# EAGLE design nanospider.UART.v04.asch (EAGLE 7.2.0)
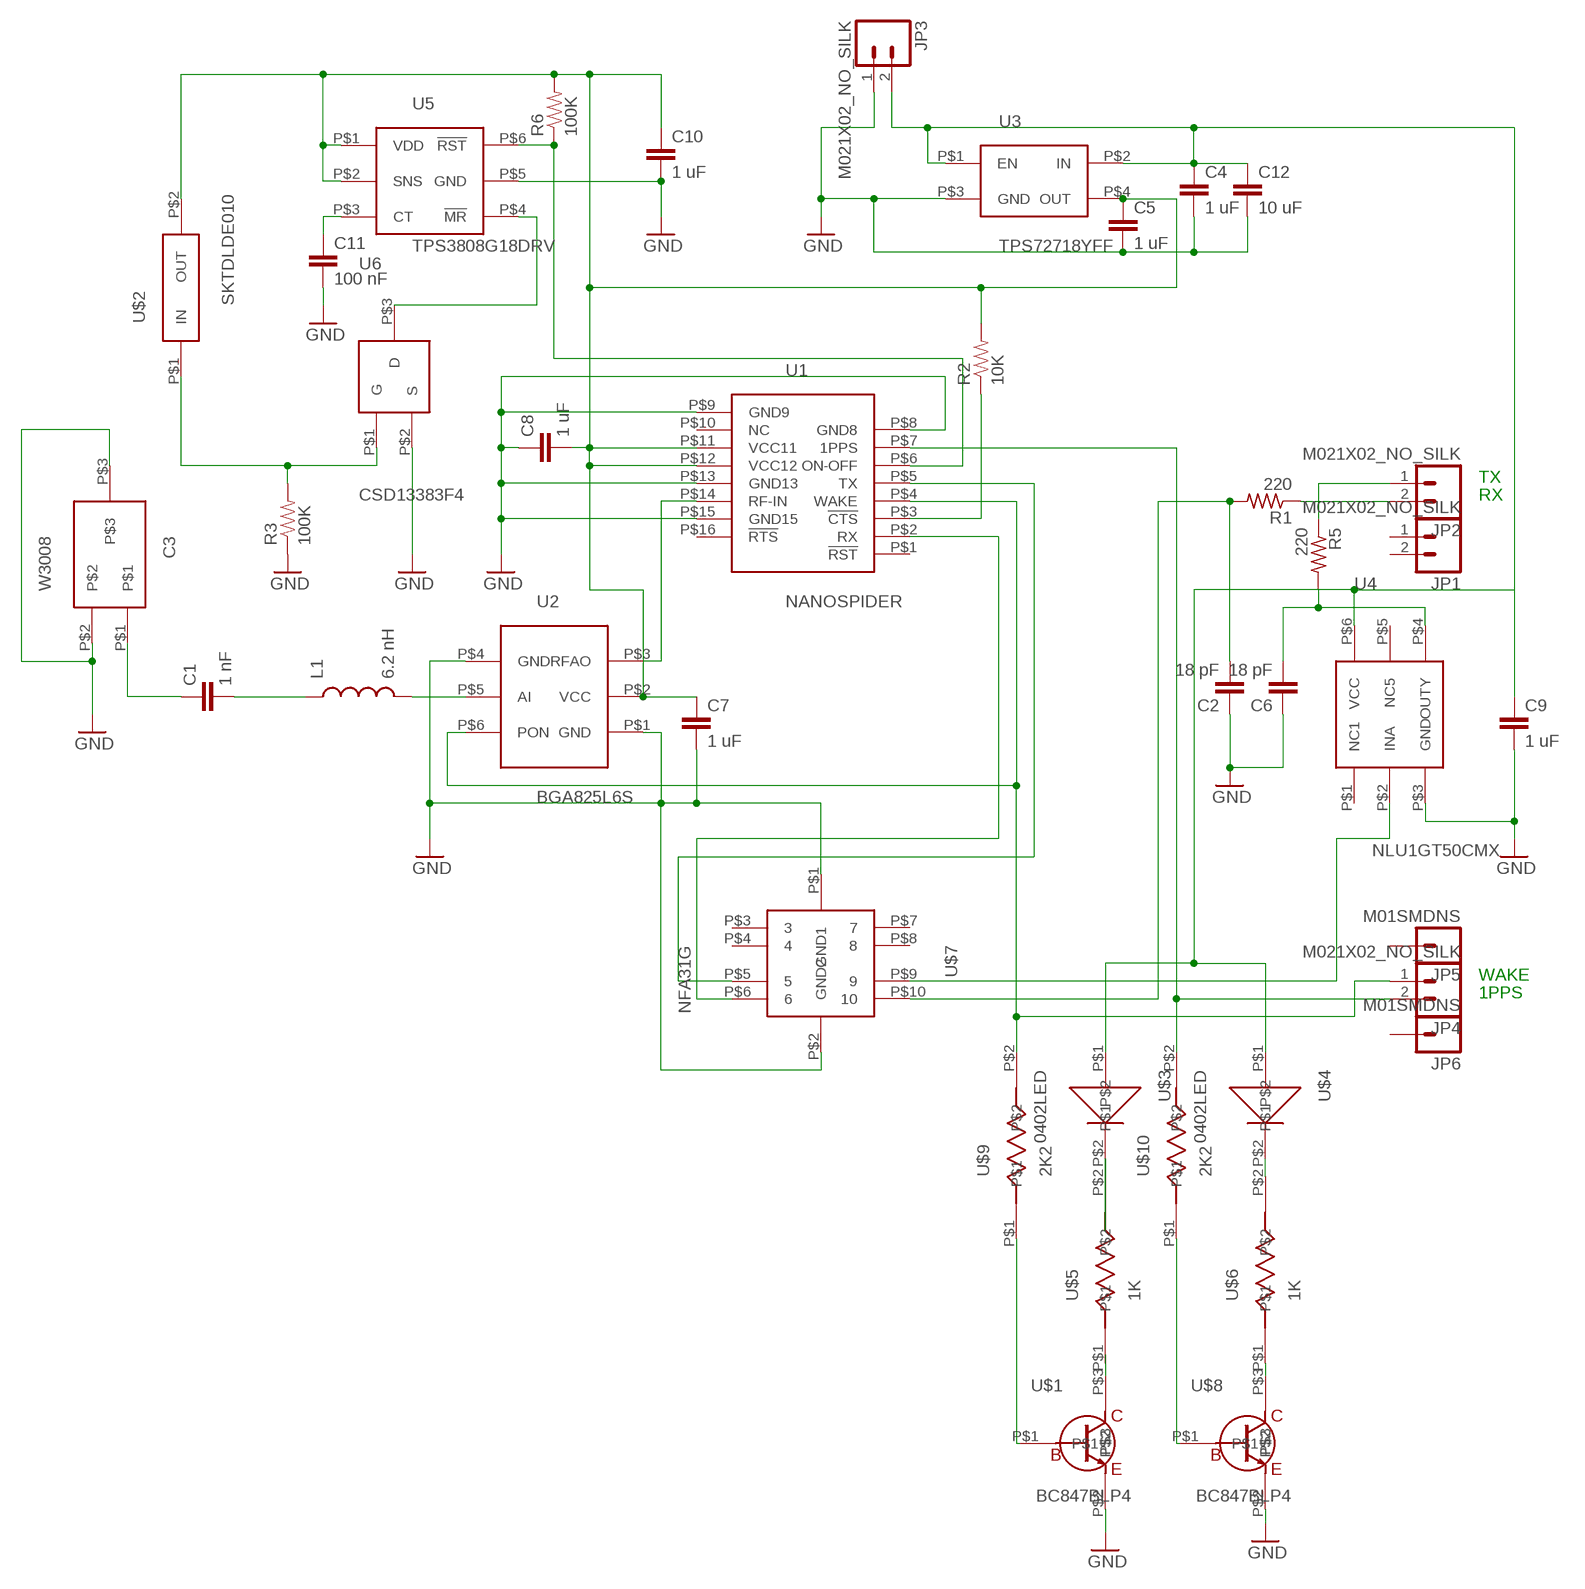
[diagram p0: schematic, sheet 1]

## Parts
C1  1 nF  0402CAP.KW  [0402-CAP]
C2  18 pF  C-EUC0402  [C0402]
C3  W3008  [W008]
C4  1 uF  0402CAP.KW  [0402-CAP]
C5  1 uF  0402CAP.KW  [0402-CAP]
C6  18 pF  C-EUC0402  [C0402]
C7  1 uF  0402CAP.KW  [0402-CAP]
C8  1 uF  0402CAP.KW  [0402-CAP]
C9  1 uF  0402CAP.KW  [0402-CAP]
C10  1 uF  0402CAP.KW  [0402-CAP]
C11  100 nF  0402CAP.KW  [0402-CAP]
C12  10 uF  0402CAP.KW  [0402-CAP]
JP1  M021X02_NO_SILK  [1X02_NO_SILK]
JP2  M021X02_NO_SILK  [1X02_NO_SILK]
JP3  M021X02_NO_SILK  [1X02_NO_SILK]
JP4  M021X02_NO_SILK  [1X02_NO_SILK]
JP5  M01SMDNS  [1X01NS]
JP6  M01SMDNS  [1X01NS]
L1  6.2 nH  INDUCTOR0402  [C0402]
R1  220  R-US_R0402  [R0402]
R2  10K  0402RES.KW  [0402-RES]
R3  100K  0402RES.KW  [0402-RES]
R5  220  R-US_R0402  [R0402]
R6  100K  0402RES.KW  [0402-RES]
U1  NANOSPIDER  [NANOSPIDER]
U2  BGA825L6S  [BGA825L6S]
U3  TPS72718YFF  [YFF0004]
U4  NLU1GT50CMX  [ULLGA6]
U5  TPS3808G18DRV  [PWSON-N6]
U6  CSD13383F4  [CSD13383F4]
U$1  BC847BLP4  [DFN1006]
U$2  SKTDLDE010  [SKTDLDE010]
U$3  0402LED  [0402LED]
U$4  0402LED  [0402LED]
U$5  1K  0402RESISTOR  [0402RESISTOR]
U$6  1K  0402RESISTOR  [0402RESISTOR]
U$7  NFA31G  [NFA31G]
U$8  BC847BLP4  [DFN1006]
U$9  2K2  0402RESISTOR  [0402RESISTOR]
U$10  2K2  0402RESISTOR  [0402RESISTOR]

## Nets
GND: C2.1 C3.P$2 C3.P$3 C4.2 C5.2 C6.1 C7.2 C8.1 C9.2 C10.2 C11.2 C12.2 JP3.1 R3.1 U1.P$8(GND8) U1.P$9(GND9) U1.P$13(GND13) U1.P$15(GND15) U2.P$1(GND) U2.P$4(GNDRF) U3.P$3(GND) U4.P$3(GND) U5.P$5(GND) U6.P$2(S) U$1.P$2 U$7.P$1(GND1) U$7.P$2(GND2) U$8.P$2
N$1: C1.1 C3.P$1
N$2: C1.2 L1.1
N$3: L1.2 U2.P$5(AI)
N$4: U1.P$14(RF-IN) U2.P$3(AO)
N$6: JP2.2 R1.1
N$7: U1.P$2(RX) U$7.P$6
N$8: U4.P$2(INA) U$7.P$9
N$9: C2.2 R1.2 U$7.P$10
N$10: C4.1 C9.1 C12.1 JP3.2 U3.P$1(EN) U3.P$2(IN) U4.P$6(VCC) U$3.P$1 U$4.P$1
N$11: C5.1 C7.1 C8.2 C10.1 R2.2 R6.2 U1.P$11(VCC11) U1.P$12(VCC12) U2.P$2(VCC) U3.P$4(OUT) U5.P$1(VDD) U5.P$2(SNS) U$2.P$2(OUT)
N$12: R3.2 U6.P$1(G) U$2.P$1(IN)
N$13: C11.1 U5.P$3(CT)
N$14: JP2.1 R5.1
N$15: U1.P$5(TX) U$7.P$5
N$16: U$1.P$1 U$9.P$1
N$17: R6.1 U1.P$6(ON-OFF) U5.P$6(!RST)
N$18: U5.P$4(!MR) U6.P$3(D)
N$19: U$1.P$3 U$5.P$1
N$20: U$3.P$2 U$5.P$2
N$21: U$8.P$1 U$10.P$1
N$22: JP4.1 U1.P$4(WAKE) U2.P$6(PON) U$9.P$2
N$23: U$6.P$1 U$8.P$3
N$27: C6.2 R5.2 U4.P$4(OUTY)
N$29: JP4.2 U1.P$7(1PPS) U$10.P$2
N$32: U$4.P$2 U$6.P$2
N$33: R2.1 U1.P$3(!CTS)
Unconnected: JP1.1 JP1.2 JP5.1 JP6.1 U1.P$1(!RST) U1.P$10(NC) U1.P$16(!RTS) U4.P$1(NC1) U4.P$5(NC5) U$7.P$3 U$7.P$4 U$7.P$7 U$7.P$8

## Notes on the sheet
- TX
- RX
- WAKE
- 1PPS

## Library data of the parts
C1 C4 C5 C7-C12 = SparkFun-Capacitors:0402CAP.KW
C2 C6 = rcl:C-EU: CAPACITOR, European symbol
C3 = Kris:W3008: W3008 2.4 GHz ceramic antenna
JP1-JP4 = SparkFun-Connectors:M02: Standard 2-pin 0.1" header. Use with
JP5 JP6 = SparkFun-Connectors:M01: Header 1
L1 = SparkFun-Passives:INDUCTOR: Inductors
R1 R5 = rcl:R-US_: RESISTOR, American symbol
R2 R3 R6 = SparkFun-Resistors:0402RES.KW
U1 = Kris:NANOSPIDER: Origin Nano Spider 4 mm x 4 mm GPS module
U2 = Kris:BGA825L6S: Infineon BGA 825L6S 1.8 V BGA amplifier for GNSS
U3 = Kris:TPS72718YFF: TI's TPS72718YFF 1.8 V RF voltage regulator
U4 = Kris:NLU1GT50CMX: NLU1GT50CMX non-inverting buffer
U5 = Kris:TPS3808G18DRV: PWSON-N6 package for TI's TPS3808G18DRV Supervisory Circuit
U6 = Kris:CSD13383F4: TI's CSD13383F4 12V N-Channel FemtoFet MOSFET
U$1 U$8 = Kris:BC847BLP4: DFN1006 package for BC847BLP4 45 V small signal NPN transistor
U$2 = Kris:SKTDLDE010: ALPS SKTDLDE010 side-mount tac switch
U$3 U$4 = Kris:0402LED: 0402led
U$5 U$6 U$9 U$10 = Kris:0402RESISTOR: 0402 resistor
U$7 = Kris:NFA31G

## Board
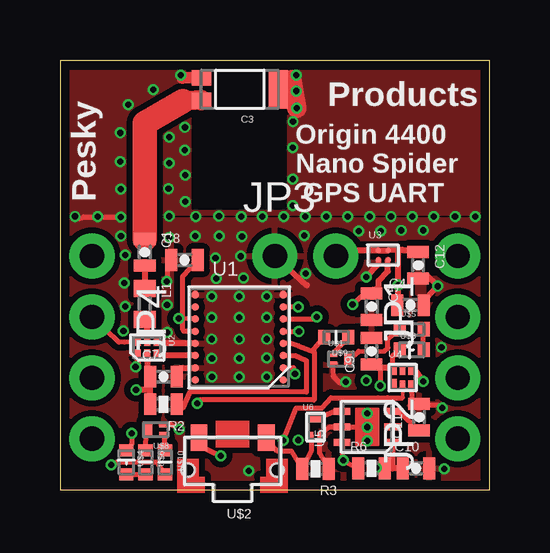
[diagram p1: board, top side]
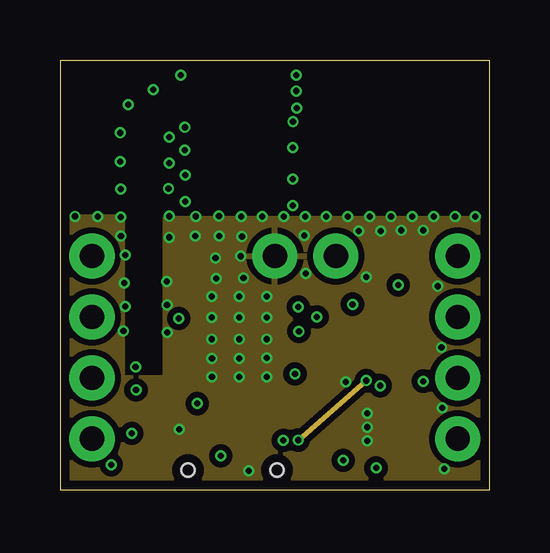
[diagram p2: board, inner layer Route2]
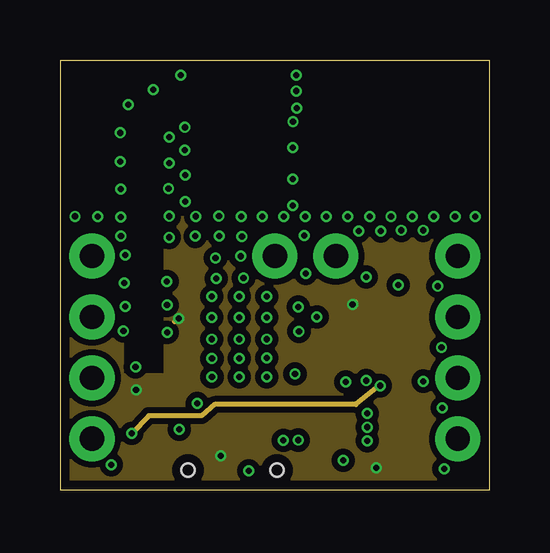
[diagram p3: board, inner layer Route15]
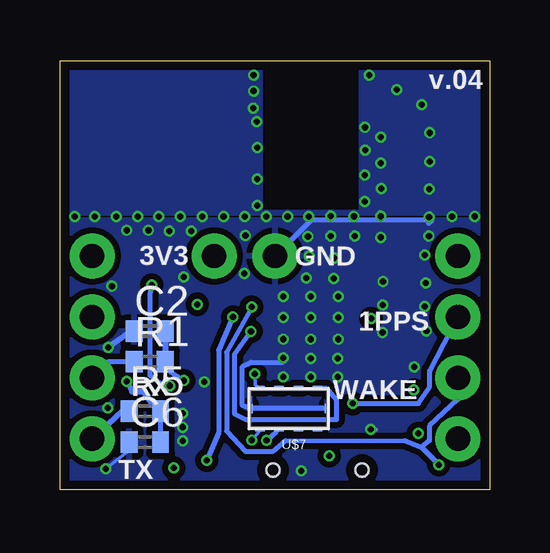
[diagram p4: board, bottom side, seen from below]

Size 17.91 x 17.9 mm. Coordinates in mm from the lower left corner, seen from the top.
Outline: 0,0 17.91,0 17.91,17.9 0,17.9 0,0
Copper layers (1*2*15*16): Top 0.035559375mm / dielectric 0.17018125mm / Route2 0.01778125mm / dielectric 47mil / Route15 0.01778125mm / dielectric 0.17018125mm / Bottom 0.035559375mm
Design rules "OSHPark-4layer *": minimum track width 5mil, minimum drill 10mil, track to track 5mil, track to pad 5mil, pad to pad 5mil, via to via 5mil, smd to smd 5mil, copper to edge 15mil, drill to drill 6mil, minimum pad ring 4mil, minimum via ring 4mil, stop-mask expansion 4mil, vias tented up to drill 20mil, thermal gap 10mil

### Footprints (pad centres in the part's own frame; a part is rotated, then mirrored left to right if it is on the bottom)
0402-CAP = smd 0.5 x 0.9: 1 -0.55,0; 2 0.55,0
C0402 = smd 0.7 x 0.9: 1 -0.65,0; 2 0.65,0
W008 = smd 0.8 x 0.65: P$1 1.6,0.475; P$2 1.6,-0.475 | smd 0.8 x 1.6: P$3 -1.6,0
1X02_NO_SILK = drill 1.016 pad 1.88: 1 0,0; 2 2.54,0
1X01NS = drill 1.016 pad 1.88: 1 0,0
R0402 = smd 0.7 x 0.9: 1 -0.65,0; 2 0.65,0
0402-RES = smd 0.5 x 0.9: 1 -0.55,0; 2 0.55,0
NANOSPIDER = smd 0.305 x 0.305: P$1 1.829,-1.778; P$2 1.829,-1.27; P$3 1.829,-0.762; P$4 1.829,-0.254; P$5 1.829,0.254; P$6 1.829,0.762; P$7 1.829,1.27; P$8 1.829,1.778; P$9 -1.829,1.778; P$10 -1.829,1.27; P$11 -1.829,0.762; P$12 -1.829,0.254; P$13 -1.829,-0.254; P$14 -1.829,-0.762; P$15 -1.829,-1.27; P$16 -1.829,-1.778
BGA825L6S = smd 0.3 x 0.25: P$1 0.225,-0.4; P$2 0.225,0; P$3 0.225,0.4; P$4 -0.225,0.4; P$5 -0.225,0; P$6 -0.225,-0.4
YFF0004 = smd 0.23 x 0.23: P$1 -0.2,0.2; P$2 0.2,0.2; P$3 -0.2,-0.2; P$4 0.2,-0.2
ULLGA6 = smd 0.22 x 0.53: P$1 -0.35,-0.325 | smd 0.22 x 0.48: P$2 0,-0.35; P$3 0.35,-0.35; P$4 0.35,0.35; P$5 0,0.35; P$6 -0.35,0.35
PWSON-N6 = smd 0.3 x 0.7: P$1 -0.65,-1.05; P$2 0,-1.05; P$3 0.65,-1.05; P$4 0.65,1.05; P$5 0,1.05; P$6 -0.65,1.05
CSD13383F4 = smd 0.15 x 0.25: P$1 -0.175,-0.325; P$2 0.175,-0.325 | smd 0.5 x 0.25: P$3 0.005,0.315
DFN1006 = smd 0.4 x 0.25: P$1 -0.35,0.225; P$2 -0.35,-0.225 | smd 0.4 x 0.7: P$3 0.35,0
SKTDLDE010 = smd 0.7 x 1.1: P$1 -1.4,-0.975; P$2 1.4,-0.975 | hole 0.55: -1.85,0.375; 1.85,0.375
0402LED = smd 0.5 x 0.6: P$1 -0.5,0; P$2 0.5,0
0402RESISTOR = smd 0.5 x 0.6: P$1 -0.5,0; P$2 0.5,0
NFA31G = smd 0.2 x 0.4: P$1 -1.6,0; P$2 1.6,0 | smd 0.4 x 0.2: P$3 -0.4,-0.85; P$4 0.4,-0.85; P$5 -1.2,-0.85; P$6 1.2,-0.85; P$7 -1.2,0.85; P$8 -0.4,0.85; P$9 0.4,0.85; P$10 1.2,0.85

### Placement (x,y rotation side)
C1  3.53,9.91 270 top
C2  14.17,6.6 0 bottom
C3  7.49,16.7 180 top
C4  14.6,7.7 0 top
C5  12.98,7.64 270 top
C6  14.38,1.98 0 bottom
C7  4.31,4.71 0 top
C8  5.19,9.58 0 top
C9  12.98,5.77 90 top
C10  14.83,0.89 0 top
C11  14.96,3.02 90 top
C12  14.92,9.35 270 top
JP1  16.57,7.2 90 top
JP2  16.57,2.12 90 top
JP3  8.95,9.74 0 top
JP4  1.33,7.2 270 top
JP5  1.33,2.12 0 top
JP6  1.33,9.74 0 top
L1  3.53,7.74 270 top
R1  14.17,5.33 0 bottom
R2  4.31,3.56 180 top
R3  10.65,0.87 180 top
R5  14.38,3.28 0 bottom
R6  12.98,0.89 0 top
U1  7.47,6.35 0 top
U2  3.63,5.92 270 top
U3  13.47,9.78 0 top
U4  14.27,4.67 0 top
U5  12.8,2.62 90 top
U6  10.64,2.62 0 top
U$1  11.7,5.44 0 top
U$2  7.19,1.19 180 top
U$3  14.65,5.83 0 top
U$4  2.76,1.14 270 top
U$5  14.65,6.68 0 top
U$6  3.57,1.14 270 top
U$7  8.38,3.38 180 bottom
U$8  3.99,2.5 180 top
U$9  11.5,6.36 180 top
U$10  4.38,1.14 270 top

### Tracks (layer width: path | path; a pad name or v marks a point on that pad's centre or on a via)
GND  (via drill 0.25)
  Top 0.152: U4.P$3 14.65,4.04 | v16,0.86 16.18,0.86
  Top 0.203: 4.07,6.16 U2.P$4 | 0.79,11.3 0.98,11.37 v2.54,11.37 | C8.1 4.48,9.37 4.47,9.07 4.48,8.7 v4.46,8.68 | C4.2 15.13,7.73 15.01,7.75 | R3.1 10.82,1.52 U6.P$2 10.82,2.31 11.25,2.62 U5.P$5 | 11.5,2.59 U5.P$5 | 14.65,4.04 14.65,3.53 | 14.65,3.53 C11.2 | 14.65,3.53 15.93,3.53 v15.93,3.4 | U5.P$5 12.79,2.62 v12.8,2.61 | U$1.P$2 11.38,4.72 11.65,4.46 11.87,4.46 v11.91,4.5 | 3.24,5.16 v3.15,5.11 | U$8.P$2 4.61,2.72 v4.97,2.51
  Top 0.254: U1.P$13 4.32,6.1 4.07,6.16 | 10.29,8.52 JP3.1 | U1.P$15 5.59,5.05 4.97,5.05 4.95,4.83 C7.2 | 15.01,7.75 v15.75,8.48 15.29,8.94 | U2.P$1 3.24,5.67 3.24,5.16 | U3.P$3 13.27,9.4 v12.76,8.86
  Top 0.406: 5.11,17.16 v5.02,17.28
  Top 0.508: C3.P$2 5.11,17.16
  Top 0.813: C3.P$3 9.66,17.11 v9.87,15.9
  Bottom 0.152: C6.1 15,1.66 v16,0.86
  Bottom 0.203: 9.12,9.63 JP3.1 7.44,11.25 2.41,11.25 2.56,11.1 v2.54,11.37 | U$7.P$1 U$7.P$2 10.31,3.51 10.31,5.13 9.96,5.31 8.64,5.31 v8.61,5.49 | v15.93,3.4 15.95,3.38 | v11.91,4.5 11.92,4.51 v11.92,4.5 | v4.97,2.51 4.94,2.49 4.78,2.5
  Bottom 0.254: C2.1 15.14,6.48 v15.89,5.93 | v12.76,8.86 12.69,8.86
  other vias: 0.62,11.4 4.55,11.4 6.62,11.4 7.54,11.39 9.32,11.39 11.1,11.39 11.99,11.39 15.57,11.39 17.3,11.39 4.46,7.69 4.48,6.55 2.68,8.63 2.64,6.61 10.19,10.59 10.24,9.02 6.32,8.05 7.47,8.05 8.61,8.05 6.32,7.19 6.32,6.27 6.33,5.46 7.47,7.19 8.61,7.19 7.47,6.27 8.61,6.27 7.47,5.47 2.72,9.78 2.72,7.65 10.21,11.39 3.89,16.69 2.84,16.05 2.51,14.88 2.51,13.67 2.52,12.53 4.52,12.55 4.55,13.61 4.55,14.71 5.21,15.11 5.2,14.15 5.22,13.11 5.22,12.01 8.43,11.39 9.7,11.84 9.7,12.96 9.69,14.27 9.71,15.35 9.85,17.28 9.85,16.63 5.66,11.4 7.87,0.78 12.8,3.17 12.8,2.04 6.33,4.71 7.47,4.71 8.61,4.71 4.55,10.52 2.54,10.58 1.58,11.38 12.9,11.39 13.79,11.39 14.68,11.38 16.46,11.39 5.64,10.57 6.63,10.57 7.58,10.55 6.48,9.66 6.5,8.81 7.52,9.73 7.65,8.83 12.45,10.79 13.36,10.79 14.23,10.82 15.13,10.82
  pour Top (isolate 0.254): 17.91,11.28 17.97,-0.02 0.04,-0.02 -0.03,11.3
  pour Bottom (isolate 0.254): -0.03,11.28 17.83,11.28 17.95,-0.02 0.01,-0.02
  pour Route2 (isolate 0.254): 0,11.38 2.59,11.4 2.59,4.67 4.39,4.7 4.39,11.33 17.91,11.33 17.87,-0.02 -0.06,-0.02 -0.03,11.38
  pour Top (isolate 0.254): 0,17.93 5.46,17.93 5.46,11.66 9.46,11.66 9.46,17.93 17.91,17.93 17.91,11.43 0,11.43
  pour Bottom (isolate 0.254): 0,17.93 5.46,17.93 5.46,11.66 9.46,11.66 9.46,17.93 17.91,17.93 17.91,11.43 0,11.43
N$1
  Top 0.813: 5.11,16.21 5.88,16.26 C3.P$1
  Top 1.016: C1.1 3.53,15.29 5.11,16.21
N$2
  Top 0.254: C1.2 L1.1
N$3
  Top 0.203: 3.63,6.88 L1.2
  Top 0.254: U2.P$5 3.63,6.88
N$4
  Top 0.254: U2.P$3 4.19,5.59 4.37,5.59 U1.P$14
N$6
  Bottom 0.203: 15.11,5.33 15.9,5.33 JP2.2
  Bottom 0.254: R1.1 15.11,5.33
N$7  (via drill 0.25)
  Top 0.203: v9.79,4.83 9.78,4.98 9.73,5.08 U1.P$2
  Bottom 0.152: U$7.P$6 9.79,4.38 v9.79,4.83
N$8  (via drill 0.25)
  Top 0.152: U4.P$2 14.28,3.84
  Top 0.203: v9.31,2.06 9.84,3.4 10.92,3.4 11.3,3.83 13.25,3.83 13.64,3.84 14.28,3.84
  Bottom 0.152: U$7.P$9 8.85,2.43 v9.31,2.06
  Bottom 0.203: v9.31,2.06 8.89,2.43
N$9  (via drill 0.25)
  Route2 0.203: v9.93,2.07 v12.76,4.55
  Bottom 0.152: U$7.P$10 9.58,2.46 v9.93,2.07
  Bottom 0.203: R1.2 13.3,4.91 13.16,4.8 v12.76,4.55
  Bottom 0.254: C2.2 R1.2
N$10  (via drill 0.25)
  Top 0.152: 13.87,5.08 U4.P$6
  Top 0.203: 13.34,5.03 v13.34,4.34 | 13.87,5.08 13.87,5.6 U$3.P$1 | v2.98,2.34 2.98,1.89 U$4.P$1
  Top 0.254: 14.18,9.99 14.29,9.99 14.62,9.99 14.84,9.99 C12.1 | 14.18,9.99 U3.P$2 U3.P$1 11.73,9.98 JP3.2 | 13.87,5.08 13.37,5.08 | 13.37,5.08 13.34,5.03 | 13.37,5.08 13.07,5.08 C9.1 | C4.1 14.1,7.96 v14.1,8.53 14.1,9.91 14.18,9.99
  Route15 0.203: v13.34,4.34 13.28,4.33 12.32,3.55 6.45,3.55 5.9,3.09 3.69,3.09 v2.98,2.34
  Bottom 0.203: v14.1,8.53 14.15,8.14 14.15,4.76 13.62,4.34 v13.34,4.34
N$11  (via drill 0.25)
  Top 0.152: U5.P$1 13.88,1.94
  Top 0.203: U1.P$11 5.11,7.14 | 5.11,7.14 5.11,8.88 5.43,9.23 C8.2 | U1.P$12 5.16,6.6 5.11,6.68 5.11,7.14 | 5.11,7.14 v4.95,7.14 | C5.1 12.66,8.14 v12.19,7.73 | U5.P$2 U5.P$1 | U$2.P$2 5.79,1.86 v6.7,1.41
  Top 0.254: 12.93,8.22 C5.1 12.9,8.3 13.26,8.37 13.26,8.71 13.66,9.11 13.66,9.58 U3.P$4 | 3.75,4.16 v3.17,4.17 | U2.P$2 3.63,5.08 C7.1 3.75,4.16 | 3.75,4.16 R2.2 | U5.P$1 13.85,1.41 13.85,1.4 13.85,0.89 R6.2 C10.1 13.36,0.88 v13.17,0.9
  Route15 0.203: v4.95,7.14 4.78,7.01 | 12.32,7.85 v12.19,7.73 | v6.7,1.41 6.69,1.38
  Route15 0.254: 3.12,4.14 v3.17,4.17 3.22,4.16 | v13.17,0.9 13.21,0.9
  pour Route15 (isolate 0.254): 0,11.4 2.6,11.42 2.6,4.79 4.38,4.78 4.38,11.35 17.88,11.35 17.88,0.02 0,0.02
N$12
  Top 0.203: U6.P$1 10.47,1.59 R3.2 10.13,1.08 9.97,1.08 9.65,1.6 9.05,1.6 U$2.P$1 8.56,2.14
N$13
  Top 0.203: U5.P$3 14.12,3.27 C11.1
N$14
  Bottom 0.203: 16.56,2.13 JP2.1
  Bottom 0.254: R5.1 15.32,3.28 15.93,2.72 16.56,2.13
N$15  (via drill 0.25)
  Top 0.203: U1.P$5 v9.96,6.6
  Bottom 0.152: 7.08,4.24 7.12,4.24 U$7.P$5
  Bottom 0.203: 7.08,4.24 6.83,4.24 6.4,3.73 6.4,2.91 10.16,2.91 10.64,3.17 10.64,5.64 v9.96,6.6
N$16
  Top 0.203: U$1.P$1 11.38,5.66 U$9.P$1
N$17  (via drill 0.25)
  Top 0.152: 12.4,0.86 R6.1
  Top 0.203: 12.4,0.86 v11.8,1.22 11.75,1.31 U5.P$6 | U1.P$6 10.62,7.11 v10.71,7.2
  Bottom 0.203: v10.71,7.2 11.3,5.82 11.3,2.38 v11.8,1.22
N$18
  Top 0.203: U5.P$4 11.46,3.27 U6.P$3
N$19
  Top 0.203: U$1.P$3 12.08,5.45 12.44,5.77 13.51,5.78 13.66,5.92 13.66,6.28 U$5.P$1
N$20
  Top 0.203: U$3.P$2 15.11,6.69 U$5.P$2
N$21
  Top 0.203: U$8.P$1 4.34,1.71 U$10.P$1
N$22  (via drill 0.25)
  Top 0.203: 10.59,5.74 10.59,3.73 5.83,3.73 v5.72,3.59 | 10.59,5.74 9.93,5.99 9.62,6.1 U1.P$4 | U2.P$6 2.69,6.15 2.45,6.15 JP4.1 | 10.59,5.74 10.59,5.87 U$9.P$2
  Bottom 0.203: v5.72,3.59 2.98,3.59 2.51,4.29 2.51,4.96 JP4.1
N$23
  Top 0.203: U$6.P$1 3.59,2.46 U$8.P$3
N$27  (via drill 0.25)
  Top 0.152: 14.74,5.05 U4.P$4
  Top 0.254: 14.74,5.05 v15.14,4.52
  Bottom 0.203: R5.2 C6.2
  Bottom 0.254: v15.14,4.52 14.91,4.09 14.45,4.09 13.89,3.34 R5.2
N$29  (via drill 0.25)
  Top 0.203: v9.93,7.62 U1.P$7 | U$10.P$2 4.04,1.11 4.04,1.15 2.38,1.15 v2.13,1.04
  Bottom 0.203: v9.93,7.62 9.98,7.49 10.97,5.74 10.97,2.44 10.2,1.6 9.04,1.6 8.51,2.06 3.53,2.04 2.83,1.75 | JP4.2 1.33,3.76 2.52,2.65 2.52,2.05 2.83,1.75 | v2.13,1.04 2.16,1.08 2.83,1.75
N$32
  Top 0.203: U$4.P$2 3.59,0.65 U$6.P$2
N$33
  Top 0.203: U1.P$3 9.8,5.59 10.26,5.39 10.26,4.07 5.42,4.07 5.09,3.37 4.97,3.38 R2.1

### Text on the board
tPlace: Products | Pesky | Origin 4400 / Nano Spider / GPS UART
bPlace: v.04 | GND | 3V3 | 1PPS | WAKE | RX | TX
